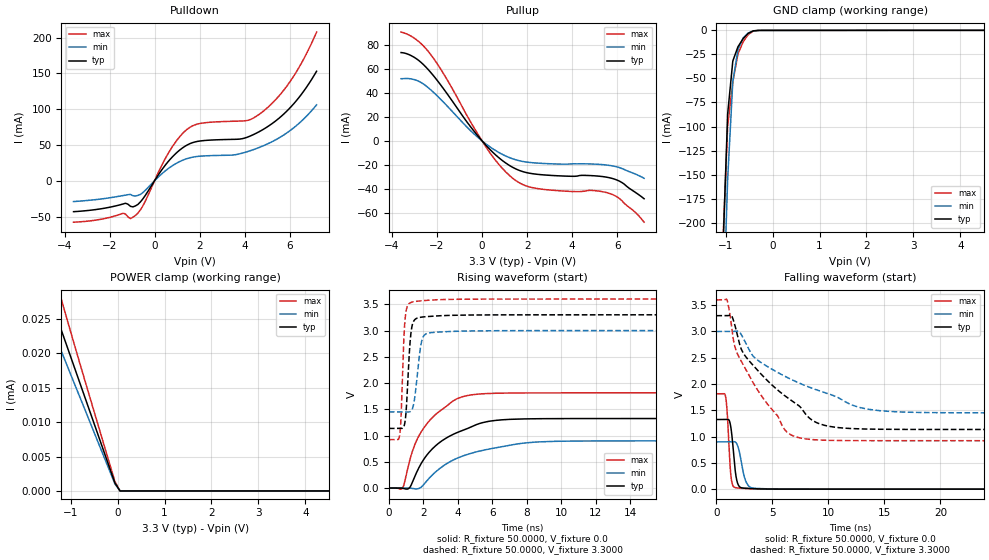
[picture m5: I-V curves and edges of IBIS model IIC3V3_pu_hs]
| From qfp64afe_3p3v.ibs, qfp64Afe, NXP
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[Model] IIC3V3_pu_hs
|   Model IIC3V3_pu_hs
| This model was characterised for following simulation conditions:
| External (pad) voltage:
|   - Typ: 3.3V,   - Min: 3.0V,   - Max: 3.6V
| Library cells for typ/min/max conditions are connected as defined below:
|  IO - External Pad
|  A - Core Input
|  EN - Output Buffer Enable
|  BOOST - vdde
|  EGP - vdd
|  EHS - vdd
|  ENZI - vdd
|  EPD - gnd
|  EPUN - gnd
|  ZI - NC
|  ZIF - NC
|  gnd - gnd
|  gnde - gnde
|  vdd - vdd
|  vdde - vdde
| All other pins connected to ground
Model_type I/O
Polarity   Non-Inverting
Enable   Active-Low
Vinl =   0.9900V
Vinh =   2.3100V
Vmeas =  1.6500V
Cref =   0.0F
Rref =   1.0000k
Vref =   0.0V
C_comp   3.5867pF   3.4362pF   3.7352pF
|C_comp_pullup   0.9045pF   0.8909pF   0.9077pF
|C_comp_pulldown   2.3321pF   2.4858pF   2.1859pF
[Model Spec]
| variable   typ   min   max
Vinh   0.9900V   0.9000V   1.0800V
Vinl   2.3100V   2.1000V   2.5200V
Vmeas   1.6500V   1.5000V   1.8000V
[Temperature Range]   25.0000   0.1250k   -40.0000
[Voltage Range]   3.3000V   3.0000V   3.6000V
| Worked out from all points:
|   slope of the pulldown table from 0 to 0.495 V, typ, clamps not added: 22 ohm
|   slope of the pullup table from 0 to 0.495 V, typ, clamps not added: 50.2 ohm
|   GND clamp passes 1 mA (typ) near -0.43 V on its own axis
|   rising waveform, R_fixture 50.0000, V_fixture 0.0: 20-80 % time 2.41ns typ, 3.15ns min, 1.81ns max; typ from 0.001 V to 1.32 V
|   rising waveform, R_fixture 50.0000, V_fixture 3.3000: 20-80 % time 230ps typ, 322ps min, 185ps max; typ from 1.14 V to 3.3 V
|   falling waveform, R_fixture 50.0000, V_fixture 0.0: 20-80 % time 371ps typ, 535ps min, 282ps max; typ from 1.32 V to 0.001 V
|   falling waveform, R_fixture 50.0000, V_fixture 3.3000: 20-80 % time 5.52ns typ, 7.85ns min, 3.83ns max; typ from 3.3 V to 1.14 V
[Pulldown]
|Voltage   I(typ)   I(min)   I(max)
-3.6V     -43.22mA   -29.09mA   -57.9mA
-1.29V    -31.46mA   -20.15mA   -46.47mA
-1.07V    -35.79mA   -19.19mA   -52.9mA
-850mV    -35.14mA   -21.36mA   -48.43mA
-520mV    -25.35mA   -16.52mA   -35.11mA
580mV     25.81mA    16.3mA     36.8mA
1.24V     45.79mA    28.53mA    65.82mA
1.9V      54.89mA    33.9mA     79.08mA
4.1V      60.55mA    40.38mA    84.05mA
4.76V     70.44mA    47.87mA    95.32mA
6.08V     103.9mA    71.39mA    141.2mA
7.2V      152.9mA    106mA      207.6mA
[Pullup]
|Voltage   I(typ)   I(min)   I(max)
-3.6V     73.65mA    51.83mA    90.73mA
-2.92V    68.52mA    50.55mA    84.41mA
-2.26V    56.61mA    42.22mA    71.46mA
-1.6V     40.53mA    30.04mA    52.53mA
160mV     -3.402mA   -2.371mA   -4.704mA
820mV     -15.2mA    -10.46mA   -21.22mA
1.37V     -22.16mA   -15.02mA   -31.28mA
1.81V     -25.65mA   -17.18mA   -36.45mA
2.47V     -27.92mA   -18.56mA   -39.79mA
5.66V     -30.76mA   -20.47mA   -43.83mA
6.1V      -33.55mA   -22.29mA   -48.04mA
7.2V      -48.27mA   -31.2mA    -67.83mA
[GND_clamp]
|Voltage   I(typ)   I(min)   I(max)
-3.6V     -5.602A    -5.487A    -5.717A
-1.07V    -242.1mA   -316.8mA   -230.6mA
-960mV    -86.82mA   -154.8mA   -99.57mA
-850mV    -31.89mA   -53.14mA   -53.6mA
-740mV    -17.03mA   -19.92mA   -24.52mA
-630mV    -8.661mA   -7.977mA   -11.97mA
-520mV    -3.068mA   -2.784mA   -4.278mA
-410mV    -504.1uA   -552.6uA   -671.9uA
7.2V      0A         0A         0A
[POWER_clamp]
|Voltage   I(typ)   I(min)   I(max)
-3.6V     71.92uA    60.65uA    145.6uA
-1.71V    33.28uA    28.87uA    40.89uA
-1.6V     31.13uA    27.02uA    37.92uA
-1.49V    28.99uA    25.16uA    35.04uA
-1.38V    26.85uA    23.31uA    32.26uA
-1.27V    24.71uA    21.46uA    29.54uA
-1.16V    22.58uA    19.61uA    26.88uA
-720mV    14.02uA    12.19uA    16.54uA
-60mV     1.171uA    1.025uA    1.377uA
50mV      0A         0A         0A
7.2V      0A         0A         0A
[Ramp]
| variable   typ   min   max
dV/dt_r  0.7945/2.4136n   0.5394/3.1455n   1.0879/1.8054n
dV/dt_f  1.2984/5.5197n   0.9292/7.8469n   1.6064/3.8342n
R_load = 50.0000
[Rising Waveform]
R_fixture= 50.0000
V_fixture= 0.0
V_fixture_min= 0.0
V_fixture_max= 0.0
|time   V(typ)   V(min)   V(max)
0s        903.5uV    965.2uV    889.6uV
783ps     -1.62mV    1.013mV    -2.423mV
1.199ns   7.692mV    -197.1uV   519.4mV
1.76ns    401.7mV    -4.517mV   1.007V
2.598ns   773.5mV    275.7mV    1.37V
3.628ns   1.008V     517.6mV    1.638V
5.429ns   1.246V     717.9mV    1.796V
7.453ns   1.315V     841.6mV    1.812V
17.61ns   1.325V     899.7mV    1.814V
1us       1.325V     899.9mV    1.814V
[Rising Waveform]
R_fixture= 50.0000
V_fixture= 3.3000
V_fixture_min= 3.0000
V_fixture_max= 3.6000
|time   V(typ)   V(min)   V(max)
0s        1.136V     1.451V     922.6mV
627.2ps   1.136V     1.451V     1.012V
700.6ps   1.135V     1.452V     1.327V
903.4ps   1.209V     1.451V     3.07V
1.101ns   2.058V     1.449V     3.486V
1.224ns   2.767V     1.455V     3.527V
1.357ns   3.107V     1.508V     3.543V
2.022ns   3.261V     2.9V       3.571V
4.424ns   3.295V     2.991V     3.598V
1us       3.3V       3V         3.6V
[Falling Waveform]
R_fixture= 50.0000
V_fixture= 0.0
V_fixture_min= 0.0
V_fixture_max= 0.0
|time   V(typ)   V(min)   V(max)
0s        1.325V     899.9mV    1.814V
822.1ps   1.325V     899.9mV    1.76V
972.8ps   1.327V     899.9mV    1.431V
1.253ns   1.223V     899.8mV    350.6mV
1.477ns   817.4mV    901.9mV    65.62mV
1.725ns   279.4mV    891.1mV    28.55mV
2.018ns   58.48mV    739.7mV    20.66mV
2.751ns   15.84mV    97.89mV    11.89mV
4.277ns   4.182mV    8.399mV    2.518mV
1us       903.5uV    965.2uV    889.6uV
[Falling Waveform]
R_fixture= 50.0000
V_fixture= 3.3000
V_fixture_min= 3.0000
V_fixture_max= 3.6000
|time   V(typ)   V(min)   V(max)
0s        3.3V       3V         3.6V
920.9ps   3.299V     3V         3.608V
1.37ns    3.295V     3V         3.071V
1.893ns   2.915V     3.01V      2.567V
2.698ns   2.498V     2.747V     2.247V
6.144ns   1.772V     2.144V     1.121V
8.74ns    1.288V     1.905V     940.8mV
10.97ns   1.17V      1.731V     926mV
23.34ns   1.136V     1.452V     922.7mV
1us       1.136V     1.451V     922.6mV
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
